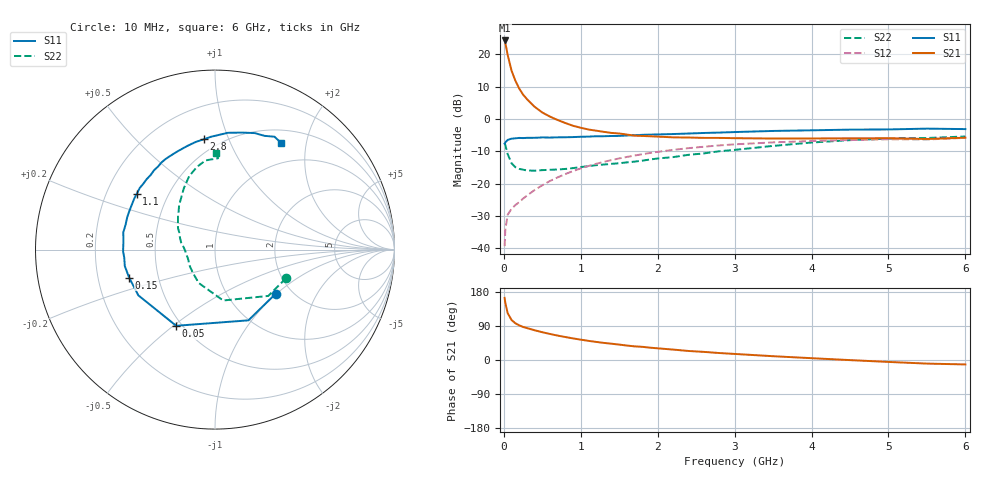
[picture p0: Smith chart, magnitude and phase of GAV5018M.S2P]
! Infineon Technologies  Discrete & RF Semiconductors
! BF775
! Si NPN RF Bipolar Junction Transistor in SOT23
! VCE = 0.5 V  IC = 18 mA
! Common Emitter S-Parameters:  May  1996
# GHz  S  MA  R  50
!  f  S11  S21  S12  S22
! GHz  MAG  ANG  MAG  ANG  MAG  ANG  MAG  ANG
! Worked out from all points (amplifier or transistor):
!   36 points, 10 MHz to 6 GHz, reference 50 ohm
!   highest |S21| = 24.3 dB at 10 MHz (marker M1)
!   |S21| within 3 dB of that: start of sweep to 37.86 MHz
!   unconditionally stable (mu >= 1): start of sweep to end of sweep
!   at 250 MHz: K = 2.66, MAG = 9.0 dB, |S12| = -24.6 dB
!   at 1.4 GHz: K = 2.55, MAG = -2.7 dB, |S12| = -12.7 dB
!   at 6 GHz: K = 1.19, MAG = -2.6 dB, |S12| = -5.8 dB
!   S11 on the Smith chart (normalised r, x): 10 MHz: 1.66, -0.99; 50 MHz: 0.47, -0.51; 150 MHz: 0.34, -0.14; 1.1 GHz: 0.33, +0.29; 2.8 GHz: 0.41, +0.82; 6 GHz: 0.68, +1.58
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0.01  0.418 -35.9  16.44 163.8  0.0108 69.6  0.4268 -21.9
0.02  0.4359 -64.7  14.96 149.9  0.0197 62.1  0.3933 -41.0
0.05  0.4764 -117.0  9.819 123.6  0.0331 45.6  0.2872 -80.9
0.1  0.4974 -149.2  5.617 105.6  0.041 40.6  0.2071 -115.9
0.15  0.5033 -161.9  3.922 96.9  0.0467 43.5  0.1798 -132.6
0.2  0.5108 -169.7  2.963 91.4  0.052 47.1  0.1693 -144.3
0.25  0.5076 -175.0  2.392 87.2  0.0587 49.9  0.1648 -152.4
0.3  0.5122 -178.8  2.037 84.3  0.0655 52.7  0.1601 -156.7
0.4  0.5127 174.2  1.549 78.5  0.0798 56.3  0.1588 -164.1
0.5  0.5199 169.4  1.263 73.3  0.0946 58.3  0.1621 -170.2
0.6  0.5171 164.4  1.09 68.7  0.1102 59.2  0.1642 -174.2
0.7  0.5213 159.7  0.966 64.4  0.1253 59.3  0.1657 -177.1
0.9  0.526 152.3  0.787 57.0  0.1571 58.2  0.1743 176.2
1.1  0.5351 144.6  0.689 50.5  0.1876 56.3  0.1873 170.9
1.3  0.5424 137.5  0.634 45.1  0.2178 53.5  0.1978 165.2
1.7  0.5614 124.3  0.554 36.0  0.2727 47.5  0.2197 154.8
2.2  0.5864 110.5  0.521 27.5  0.3335 39.0  0.2579 143.1
2.8  0.6178 95.8  0.511 18.4  0.3909 28.9  0.3178 129.0
3.5  0.6547 83.7  0.5 10.0  0.4357 18.0  0.3843 116.8
4.5  0.686 71.1  0.504 -0.3  0.4736 5.0  0.4718 102.3
5.5  0.7109 62.2  0.492 -9.5  0.4832 -6.3  0.5094 88.0
6  0.6992 58.2  0.515 -11.7  0.5111 -9.7  0.5376 89.7
